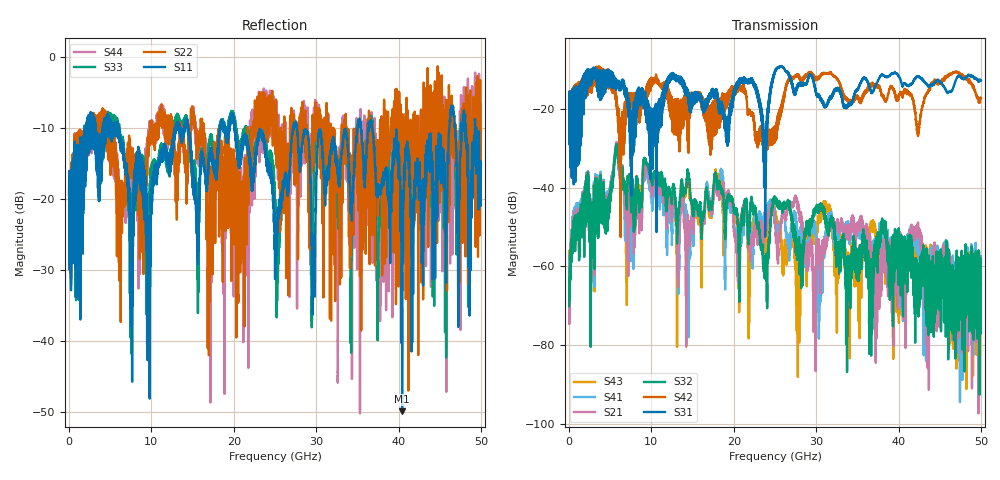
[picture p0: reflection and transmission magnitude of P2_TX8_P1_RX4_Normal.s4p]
!Keysight Technologies,N5225B,MY57041031,A.13.20.10
!Date: Friday, May 31, 2019 11:20:22
!Correction: S11(Full 4 Port(1,2,3,4))
!S12(Full 4 Port(1,2,3,4))
!S13(Full 4 Port(1,2,3,4))
!S14(Full 4 Port(1,2,3,4))
!S21(Full 4 Port(1,2,3,4))
!S22(Full 4 Port(1,2,3,4))
!S23(Full 4 Port(1,2,3,4))
!S24(Full 4 Port(1,2,3,4))
!S31(Full 4 Port(1,2,3,4))
!S32(Full 4 Port(1,2,3,4))
!S33(Full 4 Port(1,2,3,4))
!S34(Full 4 Port(1,2,3,4))
!S41(Full 4 Port(1,2,3,4))
!S42(Full 4 Port(1,2,3,4))
!S43(Full 4 Port(1,2,3,4))
!S44(Full 4 Port(1,2,3,4))
!S4P File: Measurements: <S11,S12,S13,S14>,
!<S21,S22,S23,S24>,
!<S31,S32,S33,S34>,
!<S41,S42,S43,S44>:
# Hz S  dB  R 50.0
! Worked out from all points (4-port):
!   5000 points, 10 MHz to 50 GHz, reference 50 ohm
!   strongest paths, dB at 10 MHz, 12.51 GHz, 25.01 GHz, 37.51 GHz, 50 GHz:
!     S31: -19.4, -11.5, -10.3, -12.8, -12.8
!     S42: -19.4, -19.2, -25.6, -14.4, -17.3
!     S32: -70.1, -42.9, -42.6, -56.0, -64.5
!     S21: -66.6, -46.2, -48.3, -58.6, -75.5
!     S41: -59.1, -50.4, -47.3, -53.6, -63.5
!     S43: -56.1, -46.0, -46.8, -54.2, -76.1
!   lowest |S11| = -49.9 dB at 40.44 GHz (marker M1), VSWR 1.01, Z = 49.9 - j0.307 ohm
!   |S11| at or under -10 dB: 20.17 GHz to 27.18 GHz (7.012 GHz wide, 29.6 % of centre); 27.67 GHz to 35.04 GHz (7.37 GHz wide, 23.5 % of centre); 36.79 GHz to 46.16 GHz (9.374 GHz wide, 22.6 % of centre)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
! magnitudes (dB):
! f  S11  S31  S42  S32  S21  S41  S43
! 10 MHz  -19.4  -19.4  -19.4  -70.1  -66.6  -59.1  -56.1
! 5.75 GHz  -10.4  -14.1  -17.3  -29.1  -28.6  -28.7  -29.2
! 23.86 GHz  -13.5  -40.0  -25.6  -59.7  -49.6  -46.7  -55.6
! 24.98 GHz  -25.1  -10.8  -28.5  -42.3  -49.2  -48.7  -46.0
! 27.8 GHz  -12.0  -14.4  -11.5  -53.6  -44.1  -54.0  -67.5
! 40.44 GHz  -49.9  -14.2  -16.2  -55.2  -55.5  -58.5  -55.4
! 50 GHz  -15.2  -12.8  -17.3  -64.5  -75.5  -63.5  -76.1
